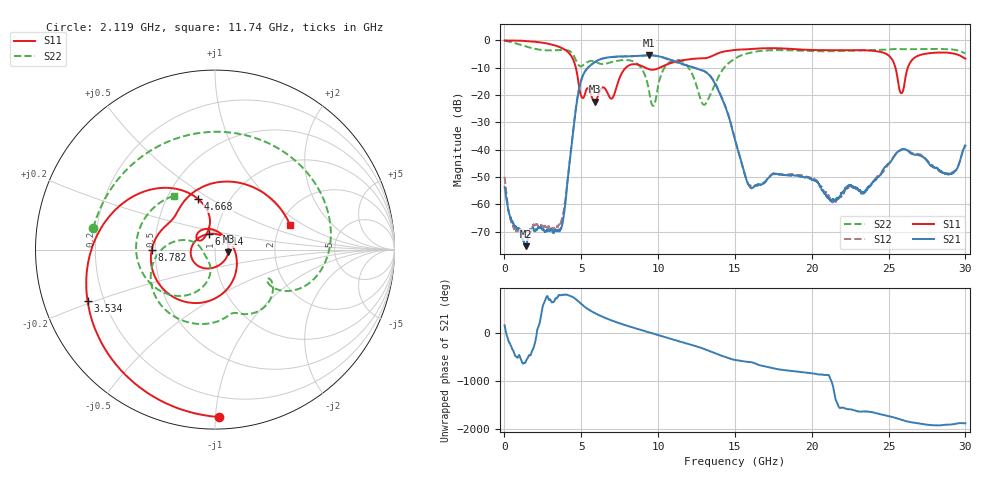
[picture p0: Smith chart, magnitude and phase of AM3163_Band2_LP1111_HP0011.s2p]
!Agilent Technologies,E8364B,MY43040894,A.07.50.67
!Agilent E8364B: A.07.50.67
!Date: Thursday, August 20, 2020 12:06:55
!Correction: S11(Full 2 Port(1,2))
!S21(Full 2 Port(1,2))
!S12(Full 2 Port(1,2))
!S22(Full 2 Port(1,2))
!S2P File: Measurements: S11, S21, S12, S22:
# Hz S  dB  R 50
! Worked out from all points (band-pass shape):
!   3201 points, 10 MHz to 30 GHz, reference 50 ohm
!   highest |S21| = -5.45 dB at 9.419 GHz (marker M1); lowest = -75.3 dB at 1.397 GHz (marker M2)
!   |S21| within 3 dB of the highest: 5.752 GHz to 11.49 GHz (5.743 GHz wide, 66.6 % of centre)
!   lowest |S11| = -22.4 dB at 5.877 GHz (marker M3), VSWR 1.16, Z = 58.1 - j1.39 ohm
!   |S11| at or under -10 dB: 4.644 GHz to 7.903 GHz (3.258 GHz wide, 51.9 % of centre); 9.165 GHz to 10.11 GHz (944 MHz wide, 9.79 % of centre); 25.45 GHz to 26.25 GHz (805.4 MHz wide, 3.12 % of centre)
!   |S22| runs from -24.0 to -0.2 dB; largest |S21 - S12| = 0.013
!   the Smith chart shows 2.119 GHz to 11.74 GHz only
!   S11 on the Smith chart (normalised r, x): 2.119 GHz: 0.07, -1.02; 3.534 GHz: 0.14, -0.19; 4.668 GHz: 0.72, +0.44; 6.814 GHz: 0.92, +0.16; 8.782 GHz: 0.48, -0.00; 11.74 GHz: 2.26, +0.77
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1e7  -0.04 -2.8  -53.68 164.3  -49.92 166.0  -0.17 -7.0
1.397038e9  -0.23 -57.5  -75.30 136.3  -70.10 162.1  -2.23 -130.6
2.118672e9  -0.60 -88.5  -69.17 36.6  -67.57 164.4  -3.24 169.8
3.533825e9  -2.31 -158.0  -69.19 74.5  -67.38 114.8  -3.55 60.0
4.667822e9  -10.56 108.4  -24.14 -16.0  -24.15 -16.4  -7.50 -32.3
5.014581e9  -20.61 123.9  -14.22 -115.8  -14.23 -116.1  -9.44 -28.6
5.876794e9  -22.43 -9.1  -7.96 60.2  -7.99 59.9  -7.75 -60.5
6.813981e9  -20.51 112.3  -6.19 -75.4  -6.23 -75.7  -8.20 -83.3
7.732425e9  -11.14 -92.1  -5.86 179.7  -5.90 179.9  -7.23 -116.5
8.782075e9  -9.05 -179.8  -5.65 76.1  -5.64 76.2  -9.30 -170.3
9.419362e9  -10.57 149.8  -5.45 14.2  -5.43 14.0  -18.78 161.2
1.000979e10  -10.24 128.9  -5.79 -44.1  -5.82 -44.7  -16.43 -101.7
1.174359e10  -7.13 18.1  -8.92 154.7  -9.00 156.5  -8.47 127.3
1.300879e10  -6.56 -50.2  -11.32 27.5  -11.27 29.0  -23.58 -103.4
1.5005e10  -3.52 -132.8  -36.39 160.0  -36.39 159.3  -6.69 -112.4
1.600779e10  -3.18 -174.5  -53.85 115.0  -53.12 118.1  -4.51 -172.8
1.787279e10  -2.91 97.8  -49.14 -38.4  -48.96 -38.2  -3.58 91.7
2.000958e10  -3.52 -10.1  -50.94 -119.3  -50.32 -121.4  -3.93 -9.8
2.230569e10  -3.56 -99.9  -53.36 -148.1  -53.99 -131.3  -3.85 -93.8
2.500479e10  -5.54 158.2  -45.04 64.2  -45.29 62.4  -3.36 -168.0
2.582952e10  -19.33 169.9  -40.06 -9.5  -39.95 -7.9  -3.22 169.5
3e10  -6.69 50.8  -38.61 -84.5  -38.13 -87.3  -4.74 54.8
